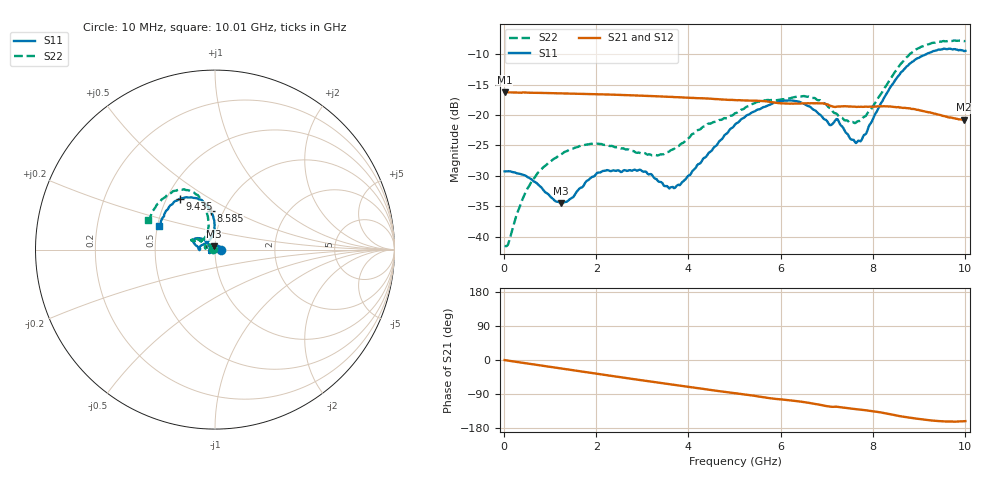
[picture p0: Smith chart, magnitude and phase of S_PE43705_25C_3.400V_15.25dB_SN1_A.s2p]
! Device ID: PE43705
! Serial: 1
! Insertion: A
! Impedance: 50 ohm
! Temp: 25C
! VDD: 3.400V
! Attenuation Step: 15.25dB
#  Hz  S  RI  R  50
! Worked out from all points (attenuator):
!   401 points, 10 MHz to 10.01 GHz, reference 50 ohm
!   highest |S21| = -16.26 dB at 10 MHz (marker M1); lowest = -20.8 dB at 9.985 GHz (marker M2)
!   lowest |S11| = -34.5 dB at 1.235 GHz (marker M3), VSWR 1.04, Z = 49.4 + j1.76 ohm
!   |S11| at or under -10 dB: start of sweep to 9.165 GHz
!   |S22| runs from -41.5 to -7.8 dB; largest |S21 - S12| = 0.0013
!   S11 on the Smith chart (normalised r, x): 10 MHz: 1.07, +0.00; 8.585 GHz: 0.87, +0.39; 9.435 GHz: 0.58, +0.37; 10.01 GHz: 0.51, +0.15
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1e7  0.0345 0.000236  0.1539 -0.000629  0.1539 -0.000606  -0.0084 0.000576
1.1e8  0.0344 0.00348  0.1533 -0.00572  0.1532 -0.00563  -0.00768 0.00523
3.35e8  0.0309 0.0113  0.1518 -0.0168  0.1517 -0.0167  -0.00948 0.0148
5.6e8  0.0242 0.0181  0.1498 -0.0276  0.1498 -0.0275  -0.0145 0.0226
1.235e9  -0.0061 0.0178  0.1391 -0.0576  0.1391 -0.0575  -0.0387 0.0276
1.685e9  -0.0246 0.00651  0.1287 -0.0757  0.1287 -0.0756  -0.0521 0.0209
2.21e9  -0.0334 -0.0105  0.1134 -0.0944  0.1133 -0.0943  -0.056 0.0103
2.96e9  -0.0298 -0.0193  0.0866 -0.1154  0.0867 -0.1153  -0.0476 0.00946
3.36e9  -0.0247 -0.0138  0.071 -0.1232  0.0712 -0.123  -0.0453 0.0124
3.835e9  -0.0266 0.0051  0.052 -0.1296  0.052 -0.1294  -0.0527 0.0241
5.01e9  -0.0619 0.0561  0.00532 -0.1326  0.00551 -0.1327  -0.0885 0.0536
5.985e9  -0.1154 0.0596  -0.0296 -0.1213  -0.0291 -0.1215  -0.1185 0.0609
6.685e9  -0.1096 0.0264  -0.0517 -0.1137  -0.0516 -0.1135  -0.1282 0.0508
7.06e9  -0.0828 0.00571  -0.0654 -0.1002  -0.065 -0.1008  -0.103 0.05
7.235e9  -0.0917 0.0112  -0.0649 -0.0978  -0.0644 -0.0975  -0.0884 0.0482
7.685e9  -0.0352 0.0505  -0.0757 -0.0892  -0.0755 -0.0894  -0.0545 0.0706
8.36e9  -0.00432 0.1639  -0.0935 -0.0713  -0.093 -0.0716  -0.0414 0.1887
8.585e9  -0.0241 0.2142  -0.0976 -0.0609  -0.0969 -0.0616  -0.0604 0.2488
8.935e9  -0.0758 0.2773  -0.1003 -0.0478  -0.1002 -0.0471  -0.1238 0.3219
9.435e9  -0.1976 0.2825  -0.0952 -0.0324  -0.0948 -0.0322  -0.2393 0.3207
9.985e9  -0.303 0.1403  -0.0869 -0.0289  -0.0864 -0.0289  -0.3632 0.1766
1.001e10  -0.3102 0.1314  -0.0872 -0.0295  -0.0871 -0.0295  -0.371 0.1655
